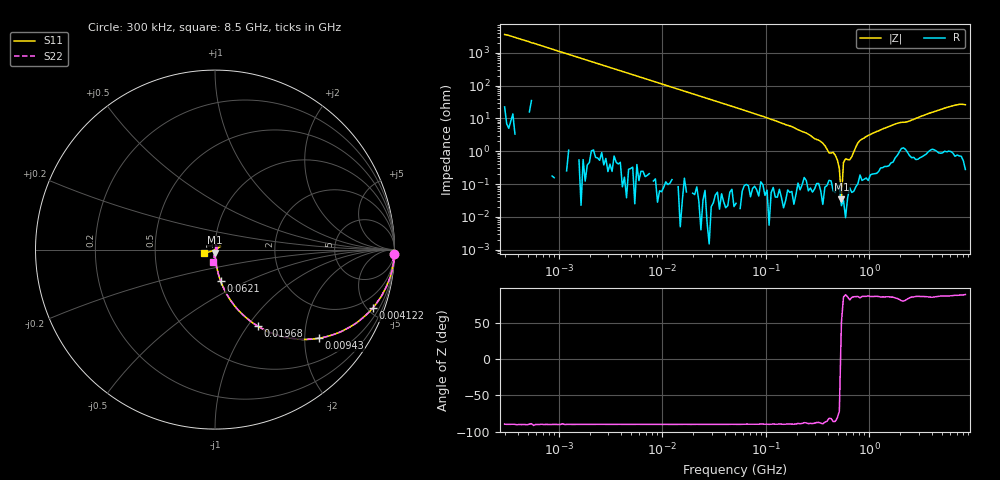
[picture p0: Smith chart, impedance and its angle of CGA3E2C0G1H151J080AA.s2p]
! S-parameter Generated by TDK Corporation
! Copyright(C) 2015 TDK Corporation.
! All Rights Reserved.
! TDK P/N: CGA3E2C0G1H151J080AA (Multilayer Ceramic Chip Capacitors)
! Property: C=150pF
! Size(LxWxT): 1.6x0.8x0.8mm, 0.063x0.031x0.031inches
! Model Type: s2p (Touchstone File Format Version 1.0)
! Frequency: DC=Yes Start=0.3MHz Stop=8500MHz 225points Log-sweep
! Note:
! Model Generated on Jun. 23, 2015
! Hash(MD5):
! Port Assignments:
!  1 ---| |--- 2
! Applicable Conditions:
!  Temperature = 25 degC
!  DC Bias Voltage = 0 V
!  Small Signal Operation
! Terms and conditions regarding TDK Simulation Models
! (1)This simulation model is being provided solely for informational purposes. Please refer to the specifications of the products in terms of detailed characteristics of such products.
! (2)In no event shall TDK Corporation of any of its subsidiaries be liable for any loss or damage arising, directly or indirectly,
!  From any information contained in this simulation model, including, but not limited to loss or damages arising from any inaccuracies, omissions or errors in connection with such information.
! (3)Any and all copyrights on this simulation model are owned by TDK Corporation.
!  Duplication or redistribution of this simulation model without prior written permission from TDK Corporation is prohibited.
! (4)This simulation model is subject to any modification or change without any prior notice.
! (5)Neither TDK Corporation nor any of its subsidiaries shall make any warranty, express or implied,
!  Including but not limited to the correctness, implied warranties of merchantability and fitness for a particular purpose with respect to this simulation models.
! (6)The use of this simulation model shall be deemed to have consented to the terms and conditions hereof.
# MHz S MA R 50
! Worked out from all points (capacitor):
!   224 points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, 300 kHz to 8.5 GHz, reference 50 ohm
!   read as one part in series: C = 144 pF near 314.1 kHz
!   lowest |Z| = 34.6 mohm at 538.9 MHz (marker M1)
!   series resonance near 536.8 MHz, so ESL is about 610 pH
!   S11 on the Smith chart (normalised r, x): 300 kHz: 1, -77; 4.122 MHz: 1.00, -5.38; 9.43 MHz: 1.00, -2.35; 19.68 MHz: 1.00, -1.13; 62.1 MHz: 1.00, -0.36; 8.5 GHz: 0.89, -0.04
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0.3  0.9996 -1.5  0.02788 88.2  0.02788 88.9  0.9996 -1.4
1.72111  0.988 -8.8  0.1536 81.2  0.1532 81.1  0.9876 -8.8
4.122422  0.9372 -20.4  0.3487 69.6  0.3487 69.6  0.9372 -20.4
9.430415  0.7616 -40.5  0.648 49.5  0.648 49.6  0.7616 -40.4
19.67787  0.4908 -60.7  0.8713 29.3  0.871 29.4  0.4906 -60.6
51.67171  0.2095 -78.1  0.9772 11.9  0.9778 11.9  0.2093 -78.1
62.1033  0.1752 -79.9  0.9829 9.9  0.9836 9.9  0.1751 -80.0
283.1228  0.03608 -87.8  0.9988 1.0  0.9986 1.1  0.03555 -88.7
538.8791  0.01662 -87.7  0.999 -1.0  0.9997 -1.0  0.01589 -95.0
778.4218  0.01003 -88.3  0.9982 -2.6  0.9972 -2.7  0.01002 -99.4
1232.735  0.002875 -90.3  0.9964 -4.9  0.9971 -5.0  0.00423 -53.9
1551.304  0.001311 -39.8  0.9953 -6.6  0.9956 -6.5  0.004381 -23.7
1952.199  0.006874 -4.1  0.9892 -8.4  0.9899 -8.3  0.01 -11.8
2140.204  0.0107 -32.8  0.9854 -8.9  0.9865 -8.9  0.01379 -33.7
3091.568  0.005144 -27.4  0.9923 -12.9  0.9932 -12.9  0.00612 -26.5
3890.506  0.01504 26.6  0.9882 -16.3  0.9891 -16.3  0.01331 27.8
5619.915  0.03526 36.0  0.9881 -23.6  0.9893 -23.5  0.03048 65.2
6754.475  0.03514 30.3  0.9886 -28.3  0.9876 -28.2  0.03053 80.8
7404.957  0.02484 30.4  0.9879 -30.9  0.987 -30.9  0.01815 74.1
7753.325  0.007541 21.3  0.9878 -32.2  0.9877 -32.3  0.002917 4.0
8118.083  0.02183 -156.2  0.9881 -33.6  0.9882 -33.7  0.02846 -98.5
8500  0.06401 -160.5  0.986 -35.2  0.9892 -35.1  0.07066 -98.1
